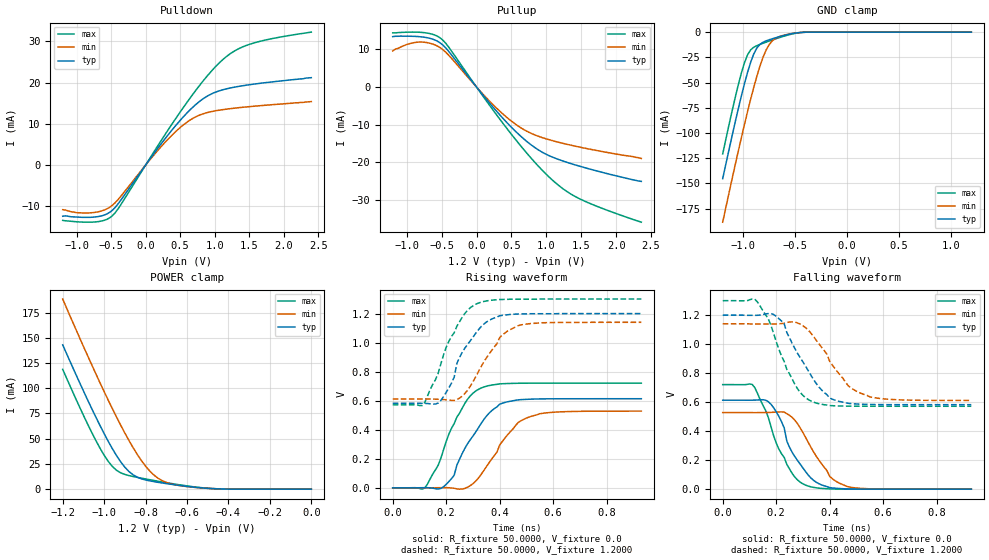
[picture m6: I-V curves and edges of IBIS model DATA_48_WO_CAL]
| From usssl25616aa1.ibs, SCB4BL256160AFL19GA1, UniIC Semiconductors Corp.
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|   Model DATA_48_WO_CAL
[Model]  DATA_48_WO_CAL
Model_type I/O
Polarity   Non-Inverting
Enable   Active-High
Vinl =   0.3800V
Vinh =   0.8200V
Vmeas =  0.6000V
Cref =   5.0000pF
Rref =   50.0000
Vref =   0.6000V
C_comp   1.7430pF   1.7110pF   1.7640pF
[Temperature Range]   25.0000   0.1250k   -40.0000
[Voltage Range]   1.2000V   1.1400V   1.3000V
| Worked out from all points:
|   slope of the pulldown table from 0 to 0.18 V, typ, clamps not added: 43.4 ohm
|   slope of the pullup table from 0 to 0.18 V, typ, clamps not added: 43.8 ohm
|   GND clamp passes 1 mA (typ) near -0.50 V on its own axis
|   POWER clamp passes 1 mA (typ) near -0.51 V on its own axis
|   rising waveform, R_fixture 50.0000, V_fixture 0.0: 20-80 % time 114ps typ, 121ps min, 102ps max; typ from 0 V to 0.614 V
|   rising waveform, R_fixture 50.0000, V_fixture 1.2000: 20-80 % time 100ps typ, 104ps min, 102ps max; typ from 0.582 V to 1.2 V
|   falling waveform, R_fixture 50.0000, V_fixture 0.0: 20-80 % time 96.3ps typ, 106ps min, 97.3ps max; typ from 0.614 V to 0 V
|   falling waveform, R_fixture 50.0000, V_fixture 1.2000: 20-80 % time 118ps typ, 121ps min, 97ps max; typ from 1.2 V to 0.582 V
[Pulldown]
|Voltage   I(typ)   I(min)   I(max)
-1.2V     -12.4mA    -10.8mA    -13.4mA
-800mV    -12.66mA   -11.57mA   -13.84mA
-600mV    -12.12mA   -10.9mA    -13.4mA
-480mV    -10.93mA   -9.725mA   -12.26mA
-360mV    -8.541mA   -7.596mA   -9.637mA
200mV     4.598mA    4.004mA    5.291mA
520mV     11.21mA    9.38mA     13.33mA
840mV     16.17mA    12.48mA    20.55mA
1.2V      18.61mA    13.64mA    26.7mA
1.4V      19.23mA    14.02mA    28.63mA
1.6V      19.72mA    14.33mA    29.77mA
2.4V      21.2mA     15.4mA     32.26mA
[Pullup]
|Voltage   I(typ)   I(min)   I(max)
-1.2V     13.4mA     9.6mA      14.4mA
-840mV    13.42mA    11.94mA    14.58mA
-680mV    13.01mA    11.71mA    14.26mA
-520mV    11.74mA    10.47mA    13.06mA
-400mV    9.531mA    8.495mA    10.66mA
80mV      -1.855mA   -1.653mA   -2.098mA
360mV     -7.948mA   -6.878mA   -9.197mA
600mV     -12.51mA   -10.42mA   -14.9mA
840mV     -16.16mA   -12.78mA   -20.12mA
1.12V     -18.88mA   -14.43mA   -25.3mA
1.4V      -20.64mA   -15.68mA   -28.99mA
2.36V     -25.1mA    -19mA      -35.95mA
[GND_clamp]
|Voltage   I(typ)   I(min)   I(max)
-1.2V     -145.3mA   -188.5mA   -120.8mA
-1.05V    -76.2mA    -118.2mA   -52.43mA
-990mV    -51.2mA    -91.62mA   -30.39mA
-960mV    -39.9mA    -78.82mA   -22.48mA
-900mV    -21.67mA   -54.7mA    -15mA
-870mV    -15.78mA   -43.66mA   -13.45mA
-810mV    -10.04mA   -24.79mA   -11.07mA
-780mV    -8.658mA   -17.59mA   -9.958mA
-720mV    -6.57mA    -8.545mA   -7.793mA
-630mV    -3.906mA   -3.64mA    -4.741mA
-420mV    -215.4uA   -240.5uA   -235uA
1.2V      1.597nA    22.84nA    1.463nA
[POWER_clamp]
|Voltage   I(typ)   I(min)   I(max)
-1.2V     143mA      188.4mA    118.7mA
-1.1V     97.38mA    141.5mA    73.24mA
-1.04V    71.38mA    114.3mA    48.22mA
-1V       55.04mA    96.69mA    33.64mA
-960mV    40mA       79.65mA    22.42mA
-900mV    21.75mA    55.6mA     14.58mA
-860mV    14.17mA    41.05mA    12.52mA
-800mV    9.133mA    22.79mA    10.12mA
-740mV    6.786mA    10.88mA    7.886mA
-660mV    4.332mA    4.436mA    5.101mA
-520mV    1.103mA    1.063mA    1.274mA
0V        1.597nA    6.003nA    2.16nA
[Ramp]
| variable   typ   min   max
dV/dt_r  0.3682/0.1099n   0.3170/0.1247n   0.4326/0.1041n
dV/dt_f  0.3705/0.1101n   0.3169/0.1297n   0.4370/99.4795p
R_load = 50.0000
[Rising Waveform]
R_fixture= 50.0000
V_fixture= 0.0
V_fixture_min= 0.0
V_fixture_max= 0.0
|time   V(typ)   V(min)   V(max)
0s        0V         0V         0V
120ps     1.127mV    174.9uV    -350.4uV
170ps     -8.205mV   946.8uV    155.4mV
220ps     63.52mV    -993.2uV   410.3mV
280ps     303.9mV    4.251mV    610.2mV
330ps     441.1mV    90.09mV    686.6mV
400ps     575.9mV    294.8mV    715.9mV
500ps     609.5mV    480.3mV    720.6mV
610ps     613.3mV    521.6mV    721mV
930ps     613.7mV    528.3mV    721mV
[Rising Waveform]
R_fixture= 50.0000
V_fixture= 1.2000
V_fixture_min= 1.1400
V_fixture_max= 1.3000
|time   V(typ)   V(min)   V(max)
0s        582.5mV    611.9mV    571.7mV
110ps     582.1mV    612.3mV    566.6mV
170ps     583.7mV    610.1mV    788.8mV
220ps     721.7mV    602.4mV    1.043V
240ps     856.5mV    608.3mV    1.113V
280ps     987.7mV    672.4mV    1.223V
320ps     1.087V     797.5mV    1.272V
400ps     1.185V     1.034V     1.297V
470ps     1.197V     1.117V     1.299V
930ps     1.2V       1.14V      1.3V
[Falling Waveform]
R_fixture= 50.0000
V_fixture= 0.0
V_fixture_min= 0.0
V_fixture_max= 0.0
|time   V(typ)   V(min)   V(max)
0s        613.7mV    528.3mV    721mV
110ps     613.6mV    527.9mV    722.3mV
170ps     603.9mV    528.9mV    498mV
200ps     534.4mV    531.5mV    318.8mV
220ps     465mV      533mV      244.3mV
240ps     330.5mV    520mV      170.6mV
310ps     120.9mV    357mV      27.87mV
400ps     10.85mV    88.56mV    1.752mV
470ps     1.473mV    15.89mV    189.9uV
930ps     0V         0V         0V
[Falling Waveform]
R_fixture= 50.0000
V_fixture= 1.2000
V_fixture_min= 1.1400
V_fixture_max= 1.3000
|time   V(typ)   V(min)   V(max)
0s        1.2V       1.14V      1.3V
130ps     1.199V     1.139V     1.291V
170ps     1.211V     1.139V     1.176V
230ps     1.14V      1.144V     880.7mV
280ps     936.5mV    1.146V     692.3mV
340ps     755.6mV    1.052V     600.1mV
400ps     629mV      882mV      576.8mV
470ps     591.8mV    712.1mV    572.4mV
520ps     585.9mV    659mV      571.9mV
930ps     582.5mV    611.9mV    571.7mV
